FUNCTION_BLOCK FB_Visu
VAR
	// ============================== 轴 NCTOPLC 的输入结构体 =====================================
	
	// 这里没用AXIS_REF是因为轴变量不能多次绑定，而 NCTOPLC_AXIS_REF 的某些状态字是可以多次绑定的，在模拟程序中，只会用到一些状态字去检测轴的一些 NC 参数
	
	MainAxisState			AT %I*		: NCTOPLC_AXIS_REF;			// 运输皮带 	NCTOPLC 的输入结构体
	MetalAxisState			AT %I*		: NCTOPLC_AXIS_REF;			// 金属分拣皮带 NCTOPLC 的输入结构体
	PlasticAxisState		AT %I*		: NCTOPLC_AXIS_REF;			// 塑料分拣皮带 NCTOPLC 的输入结构体
	bresetAxis				AT %Q*      : BOOL;						// 如果主程序当中的轴出现 NC 报错，那需要在 HMI 当中做一个按钮去复位轴报错
	
	// =================================== 设备的一些状态 ===============================
	bComprAirEnabled		AT %I*		: BOOL;						// 如果为TRUE，则设备的气缸空气被压缩
	bPowerEnabled			AT %I*		: BOOL;						// 如果为TRUE，则设备已经使能
	bClampToWork			AT %I*		: BOOL;						// 如果为TRUE，则正位气缸存在输出
	bBarrierToWork			AT %I*		: BOOL;						// 如果为TRUE，则栏杆气缸存在输出
	bMetalToWork			AT %I*		: BOOL;						// 如果为TRUE，则金属分拣气缸存在输出
	bPlasticToWork			AT %I*		: BOOL;						// 如果为TRUE，则塑料分拣气缸存在输出
	
	// ====================================== 错误信息 ====================================
	bError					AT %I*		: BOOL;						// 如果为TRUE，则设备存在错误
	bClampError				AT %I*		: BOOL;						// 如果为TRUE，则正位气缸存在错误
	sClampErrMsg			AT %I*		: STRING;					// 正位气缸的错误信息
	bMetalCylError			AT %I*		: BOOL;						// 如果为TRUE，则金属分拣气缸存在错误
	sMetalErrMsg			AT %I*		: STRING;					// 金属分拣气缸的错误信息
	bPlasticCylError		AT %I*		: BOOL;						// 如果为TRUE，则塑料分拣气缸存在错误
	sPlasticErrMsg			AT %I*		: STRING;					// 塑料分拣气缸的错误信息
	sMessageMainAxis		AT %I*		: STRING;					// 运输皮带的错误信息
	sMessageMetalAxis		AT %I*		: STRING;					// 金属分拣出料皮带的错误信息
	sMessagePlasticAxis		AT %I*		: STRING;					// 塑料分拣出料皮带的错误信息

	
	// ============================ PackML状态机的状态标志位 ==============================
	bStarted				AT %I*		: BOOL;						// 如果为TRUE，则设备在运行状态
	bStopped				AT %I*		: BOOL;						// 如果为TRUE，则设备在停止状态
	bReset					AT %I*		: BOOL;						// 如果为TRUE，则设备在复位中状态
	bAborted				AT %I*		: BOOL;						// 如果为TRUE，则设备在中止状态
	bIdle					AT %I*		: BOOL;						// 如果为TRUE，则设备在空闲状态
	bAuto					AT %I*		: BOOL;						// 如果为TRUE，则设备在自动模式
	bSemi					AT %I*		: BOOL;						// 如果为TRUE，则设备在半自动模式
	bManual					AT %I*		: BOOL;						// 如果为TRUE，则设备在手动模式
	bMaintenance			AT %I*		: BOOL;						// 如果为TRUE，则设备在维护模式
	
	bStartButtonOff			AT %I*		: BOOL;						// 自复位启动按钮的中间变量

	// ============================ HMI 按钮输入的状态 ==================================
	
	// HMI按钮信号直接传递给bButtonXXXOut，绑定给主程序信号处理功能块的In，然后经过主程序信号处理功能块的Out绑定回来，用来做一些 HMI 按钮颜色，切换的逻辑
	
	bButtonPowerIn			AT %I*		: BOOL;						// 使能按钮的状态
	bButtonComprAirIn		AT %I*		: BOOL;						// 气缸压缩按钮的状态
	bButtonStartIn			AT %I*		: BOOL;						// 启动按钮的状态
	bButtonStopIn			AT %I*		: BOOL;						// 停止按钮的状态
	bButtonResetIn			AT %I*		: BOOL;						// 复位按钮的状态
	bButtonAbortIn			AT %I*		: BOOL;						// 中止按钮的状态
	
	bButtonAutoIn			AT %I*		: BOOL;						// 自动模式按钮的状态
	bButtonSemiIn			AT %I*		: BOOL;						// 半自动模式按钮的状态
	bButtonManuIn			AT %I*		: BOOL;						// 手动模式按钮的状态
	bButtonMaintenanceIn	AT %I*		: BOOL;						// 维护模式按钮的状态

	bButtonMainFwIn			AT %I*		: BOOL;						// 正向点动输送皮带按钮的状态
	bButtonMainBwIn			AT %I*		: BOOL;						// 反向点动输送皮带按钮的状态
	bButtonMetalFwIn		AT %I*		: BOOL;						// 正向点动金属分拣出料皮带按钮的状态
	bButtonMetalBwIn		AT %I*		: BOOL;						// 反向点动金属分拣出料皮带按钮的状态
	bButtonPlasticFwIn		AT %I*		: BOOL;						// 正向点动塑料分拣出料皮带按钮的状态
	bButtonPlasticBwIn		AT %I*		: BOOL;						// 反向点动塑料分拣出料皮带按钮的状态
	
	bButtonClampToWorkIn	AT %I*		: BOOL;						// 正位气缸输出按钮的状态
	bButtonBarrierToWorkIn	AT %I*		: BOOL;						// 栏杆气缸输出按钮的状态
	bButtonMetalToWorkIn	AT %I*		: BOOL;						// 金属分拣气缸输出按钮的状态
	bButtonPlasticToWorkIn	AT %I*		: BOOL;						// 塑料分拣气缸输出按钮的状态


	
	// ============================== HMI 按钮的输出信号 ===============================
	
	// 绑定给主程序信号处理功能块的In
	
	bButtonPowerOut			AT %Q*		: BOOL;						// 使能按钮的信号
	bButtonComprAirOut		AT %Q*		: BOOL;						// 气缸压缩按钮的信号
	bButtonStartOut			AT %Q*		: BOOL;						// 启动按钮的信号
	bButtonStopOut			AT %Q*		: BOOL;						// 停止按钮的信号
	bButtonResetOut			AT %Q*		: BOOL;						// 复位按钮的信号
	
	bButtonAutoOut			AT %Q*		: BOOL;						// 自动模式按钮的信号	
	bButtonSemiOut			AT %Q*		: BOOL;						// 半自动模式按钮的信号
	bButtonManuOut			AT %Q*		: BOOL;						// 手动模式按钮的信号
	bButtonMaintenanceOut	AT %Q*		: BOOL;						// 维护模式按钮的信号	
	
	bButtonMainFwOut		AT %Q*		: BOOL;						// 正向点动输送皮带按钮的信号
	bButtonMainBwOut		AT %Q*		: BOOL;						// 反向点动输送皮带按钮的信号
	bButtonMetalFwOut		AT %Q*		: BOOL;						// 正向点动金属分拣出料皮带按钮的信号
	bButtonMetalBwOut		AT %Q*		: BOOL;						// 反向点动金属分拣出料皮带按钮的信号
	bButtonPlasticFwOut		AT %Q*		: BOOL;						// 正向点动塑料分拣出料皮带按钮的信号
	bButtonPlasticBwOut		AT %Q*		: BOOL;						// 反向点动塑料分拣出料皮带按钮的信号
	
	bButtonClampToWorkOut	AT %Q*		: BOOL;						// 正位气缸输出按钮的信号
	bButtonBarrierToWorkOut	AT %Q*		: BOOL;						// 栏杆气缸输出按钮的信号
	bButtonMetalToWorkOut	AT %Q*		: BOOL;						// 金属分拣气缸输出按钮的信号
	bButtonPlasticToWorkOut	AT %Q*		: BOOL;						// 塑料分拣气缸输出按钮的信号

	
	// =========================== 模拟程序当中元素的坐标参数 ===========================
	fYClamp								: LREAL;					// 正位气缸的纵坐标
	fYBarrier							: LREAL;					// 栏杆气缸的纵坐标
	fYMetal								: LREAL;					// 金属分拣气缸的纵坐标
	fYPlastic							: LREAL;					// 塑料分拣气缸的纵坐标
	aBoxX								: ARRAY[1..4] OF LREAL;		// 物料的横坐标数组
	aBoxY								: ARRAY[1..4] OF LREAL;		// 物料的纵坐标数组

	// ============================= 物料移动参数 =========================================
	nLastBox						: INT;						// 在运输皮带当中物料的序号，			如：nLastBox := 1，则一号物料在运输当中
	aBoxMetalMove					: ARRAY[1..4] OF BOOL;		// 第几个物料在被金属分拣气缸分拣，		如：aBoxMetalMove[1] := TRUE，则一号物料在被金属分拣气缸分拣
	aBoxMetalFree					: ARRAY[1..4] OF BOOL;		// 第几个物料没在被金属分拣气缸分拣		如：aBoxMetalFree[1] := TRUE，则一号物料没有在被金属分拣气缸分拣
	aBoxPlasticMove					: ARRAY[1..4] OF BOOL;		// 第几个物料在被塑料分拣气缸分拣		如：aBoxPlasticMove[1] := TRUE，则一号物料在被金属分拣气缸分拣
	aBoxPlasticFree					: ARRAY[1..4] OF BOOL;		// 第几个物料没在被塑料分拣气缸分拣		如：aBoxPlasticFree[1] := TRUE，则一号物料没有在被塑料分拣气缸分拣
	aBoxMainBelt					: ARRAY[1..4] OF BOOL;		// 第几个物料在运输皮带当中运输			如：aBoxMainBelt[1] := TRUE，则一号物料在运输当中
	aBoxMetalBelt					: ARRAY[1..4] OF BOOL;		// 第几个物料在金属分拣皮带当中运出		如：aBoxMetalBelt[1] := TRUE，则一号物料在运输当中
	aBoxPlasticBelt					: ARRAY[1..4] OF BOOL;		// 第几个物料在塑料分拣皮带当中运出		如：aBoxPlasticBelt[1] := TRUE，则一号物料在运输当中
	
	fMainVelo						: LREAL;					// 运输皮带的转动速度
	fMetalVelo						: LREAL;					// 金属分拣皮带的转动速度
	fPlasticVelo					: LREAL;					// 塑料分拣皮带的转动速度
	
	bAccident						: BOOL;						// 如果为TRUE，则出现意外事故			如：撞机
	nState							: INT;						// 物料的索引							如：nState := 1，则当前是1号物料
	
	// ================================= 信息 ==========================================
	nMessages						: INT;						// 信息的个数
	sMessageClamp					: STRING;					// 正位气缸的信息
	sMessageMetalCyl				: STRING;					// 金属分拣气缸的信息
	sMessagePlasticCyl				: STRING;					// 塑料分拣气缸的信息

	
	// ============================= 轴运动的参数 =======================================
	nAngleMain						: INT;						// 输送皮带转动时旋转的角度（HMI）
	nAngleMetal						: INT;						// 金属分拣皮带转动时旋转的角度（HMI）
	nAnglePlastic					: INT;						// 塑料分拣皮带转动时旋转的角度（HMI）
	fbTimerMainAxis					: TON;						// 输送皮带转动时到 HMI 图标开始转动的计时器 TON 功能块 
	fbTimerMetalAxis				: TON;						// 金属分拣皮带转动时到 HMI 图标开始转动的计时器 TON 功能块 
	fbTimerPlasticAxis				: TON;						// 塑料分拣皮带转动时到 HMI 图标开始转动的计时器 TON 功能块 
	tMoveAxis						: TIME := T#0MS;			// 皮带转动时到 HMI 图标开始转动的延迟时间，这里随机设置一个40ms较短的时间

	// ========================= 按钮颜色的相关参数 ====================================
	nButtonColorStart				: DWORD;					// 启动按钮的颜色
	bButtonColorStart				: BOOL;						// 如果为TRUE，则切换启动按钮的颜色
	nButtonColorStop				: DWORD;					// 停止按钮的颜色
	bButtonColorStop				: BOOL;						// 如果为TRUE，则切换停止按钮的颜色
	nButtonColorReset				: DWORD;					// 复位按钮的颜色
	bButtonColorReset				: BOOL;						// 如果为TRUE，则切换停止按钮的颜色
	nButtonColorAuto				: DWORD;					// 自动模式按钮的颜色
	bButtonColorAuto				: BOOL;						// 如果为TRUE，则切换自动模式按钮的颜色
	nButtonColorSemi				: DWORD;					// 半自动模式按钮的颜色
	bButtonColorSemi				: BOOL;						// 如果为TRUE，则切换半自动模式按钮的颜色
	nButtonColorManu				: DWORD;					// 手动模式按钮的颜色
	bButtonColorManu				: BOOL;						// 如果为TRUE，则切换手动模式按钮的颜色
	nButtonColorMaint				: DWORD;					// 维护模式按钮的颜色
	bButtonColorMaint				: BOOL;						// 如果为TRUE，则切换维护模式按钮的颜色
	nButtonColorClamp				: DWORD;					// 手动控制正位气缸按钮的颜色
	bButtonColorClamp				: BOOL;						// 如果为TRUE，则切换手动控制正位气缸按钮的颜色
	nButtonColorBarrier				: DWORD;					// 手动控制栏杆气缸按钮的颜色
	bButtonColorBarrier				: BOOL;						// 如果为TRUE，则切换手动控制栏杆气缸按钮的颜色
	nButtonColorMetalCyl			: DWORD;					// 手动控制金属分拣气缸按钮的颜色
	bButtonColorMetalCyl			: BOOL;						// 如果为TRUE，则切换金属分拣气缸按钮的颜色
	nButtonColorPlasticCyl			: DWORD;					// 手动控制塑料分拣气缸按钮的颜色
	bButtonColorPlasticCyl			: BOOL;						// 如果为TRUE，则切换塑料分拣气缸按钮的颜色
	nButtonColorMainFw				: DWORD;					// 手动控制输送皮带正转按钮的颜色
	bButtonColorMainFw				: BOOL;						// 如果为TRUE，则切换手动控制输送皮带正转按钮的颜色
	nButtonColorMainBw				: DWORD;					// 手动控制输送皮带反转按钮的颜色
	bButtonColorMainBw				: BOOL;						// 如果为TRUE，则切换手动控制输送皮带反转按钮的颜色
	nButtonColorMetalFw				: DWORD;					// 手动控制金属分拣皮带正转按钮的颜色
	bButtonColorMetalFw				: BOOL;						// 如果为TRUE，则切换手动控制金属分拣皮带正转按钮的颜色
	nButtonColorMetalBw				: DWORD;					// 手动控制金属分拣皮带反转按钮的颜色
	bButtonColorMetalBw				: BOOL;						// 如果为TRUE，则切换手动控制金属分拣皮带反转按钮的颜色
	nButtonColorPlasticFw			: DWORD;					// 手动控制塑料分拣皮带正转按钮的颜色
	bButtonColorPlasticFw			: BOOL;						// 如果为TRUE，则切换 手动控制塑料分拣皮带正转按钮的颜色
	nButtonColorPlasticBw			: DWORD;					// 手动控制塑料分拣皮带反转按钮的颜色
	bButtonColorPlasticBw			: BOOL;						// 如果为TRUE，则切换手动控制塑料分拣皮带反转按钮的颜色
	nButtonColorComprAir			: DWORD;					// 压缩气缸空气按钮的颜色
	bButtonColorComprAir			: BOOL;						// 如果为TRUE，则切换压缩气缸空气按钮的颜色

	// ================================== 其他 =======================================
	RandomGenerator					: DRAND;					// 随机函数生成的功能块
	RandomNumber					: LREAL;					// 随机数（0-1）
	bRandomChangeColor				: BOOL;						// 如果为TRUE，则随机的切换物料颜色
	ArrChangeColor					: ARRAY[1..4] OF BOOL	:= [TRUE,FALSE,FALSE,TRUE];	// 物料的随机颜色：如：ArrChangeColor[1]:= true; 则1号物料是灰色
	
	bButtonColorAutoNew				: BOOL;						// 如果为TRUE，则当前控制模式为自动模式且无报错，用来启用 HMI 当中的自动按钮
	bButtonColorSemiNew				: BOOL;						// 如果为TRUE，则当前控制模式为半自动模式且无报错，用来启用 HMI 当中的半自动按钮
	bButtonColorManuNew				: BOOL;						// 如果为TRUE，则当前控制模式为手动模式且无报错，用来启用 HMI 当中的手动按钮
	bButtonColorMaintNew			: BOOL;						// 如果为TRUE，则当前控制模式为维护模式且无报错，用来启用 HMI 当中的维护按钮
END_VAR
VAR CONSTANT
	// ================================== 颜色 =======================================
	cYellow 									: DWORD	:= 16#00FFFF80;		// 黄色的ARGB对应的16进制值
	cGreen 										: DWORD	:= 16#0080FF00;		// 绿色的ARGB对应的16进制值
	cPink 										: DWORD	:= 16#00FF8080;		// 粉色的ARGB对应的16进制值
	
	// ============================ HMI图标移动参数 ===================================
	cVelocityDenominator						: LREAL := 250.0;			// 速度比例分母。HMI 图标旋转的速度是实际轴速度的一个比值。
	cAxisMovementSemiPlusAuto					: INT 	:= 2;				// 半自动和自动模式下，HMI 轴每个PLC周期的移动角度
	cAxisMovementManual							: INT 	:= 1;				// 手动模式下，HMI 轴每个PLC周期的移动角度
	cClampMovement								: LREAL := 0.1;				// 每个PLC周期正位气缸的移动量
	cBarrierMovement							: LREAL := 1.0;				// 每个PLC周期栏杆气缸的移动量
	cMetalPlasticCylMovement					: LREAL := 1.0;				// 每个PLC周期塑料/金属分拣气缸的移动量
	
	// ========================= HMI图标各个位置的标定参数 ============================
	cYClampCylStartPos							: LREAL := 0.0;				// 正位气缸的基始位置纵坐标
	cYClampCylEndPos							: LREAL := 3.0;				// 正位气缸的目标位置纵坐标
	cYBarrierCylStartPos						: LREAL := 0.0;				// 栏杆气缸的基始位置纵坐标
	cYBarrierCylEndPos							: LREAL := 63.0;			// 栏杆气缸的目标位置纵坐标
	cYMetalPlasticCylStartPos					: LREAL := 0.0;				// 金属/塑料分拣气缸的基始位置纵坐标
	cYMetalPlasticCylEndPos						: LREAL := -73.0;			// 金属/塑料分拣气缸的目标位置纵坐标
	
	// =========================== 物料宽度、距离参数 ==================================
	cBoxWidth									: LREAL := 60.0;			// HMI 当中物料的宽度
	cBarrierWidth								: LREAL := 30.0;			// HMI 当中栏杆气缸的宽度
	cDiffBarrierToStartOfMetalCyl				: LREAL := 191.0;			// HMI 当中从栏杆气缸到金属分拣气缸左侧位置的距离，单位为像素或实际测量单位
	cDiffBarrierToEndOfMetalCyl					: LREAL := 261.0;			// HMI 当中从栏杆气缸到金属分拣气缸右侧位置的距离，单位为像素或实际测量单位
	cDiffBarrierToStartOfPlasticCyl				: LREAL := 441.0;			// HMI 当中从栏杆气缸到塑料分拣气缸左侧位置的距离，单位为像素或实际测量单位
	cYMetalPlasticCylOnMainBelt					: LREAL := -9.0;			// HMI 当中金属和塑料分拣气缸到达主传送带时的位置纵坐标
	cYBoxesOnMetalPlasticBelt_min				: LREAL := -65.0;			// HMI 当中物料在金属或塑出料皮带上时的最小位置的纵坐标
	cYBoxesOnMetalPlasticBelt_max				: LREAL := -140.0;			// HMI 当中物料在金属或塑出料皮带上时的最大位置的纵坐标
	
	// ======================== 输送皮带当中物料的距离参数 ==============================
	cYforAllBoxesOnMainBelt						: LREAL := -5.0;			// HMI 当中物料在输送皮带上的纵坐标
	cYforAllBoxesNotOnMainBelt					: LREAL := -60.0;			// HMI 当中物料不在输送皮带上的纵坐标
	
	cYforAllBoxesStartPosMainBelt				: LREAL := 0.0;				// HMI 当中物料在输送皮带的第一个位置时的纵坐标
	cXforAllBoxesStartPosMainBelt				: LREAL := -240.0;			// HMI 当中物料在输送皮带的第一个位置时的横坐标
	cXforAllBoxesLastPossiblePosMainBelt		: LREAL := 461.0;			// HMI 当中物料在输送皮带上，可以移动到的最后位置横坐标
	
	cXforAllBoxesCorrectPushMetalCyl_min		: LREAL := 180;				// HMI 当中被金属分拣气缸推到金属出料皮带时，物料最小位置的横坐标
	cXforAllBoxesCorrectPushMetalCyl_max		: LREAL := 211;				// HMI 当中被金属分拣气缸推到金属出料皮带时，物料最大位置的横坐标
	cXforAllBoxesIncorrectPushMetalCyl_min		: LREAL := 131;				// HMI 当中被金属分拣气缸推出，但未推到金属出料皮带时，物料最小位置的横坐标
	cXforAllBoxesIncorrectPushMetalCyl_max		: LREAL := 261;				// HMI 当中被金属分拣气缸推出，但未推到金属出料皮带时，物料最大位置的横坐标
	
	cXforAllBoxesCorrectPushPlasticCyl_min		: LREAL := 430;				// MMI 当中被塑料分拣气缸推到塑料出料皮带时，物料最小位置的横坐标
	cXforAllBoxesCorrectPushPlasticCyl_max		: LREAL := 461;				// HMI 当中被塑料分拣气缸推到塑料出料皮带时，物料最大位置的横坐标
	cXforAllBoxesIncorrectPushPlasticCyl_min	: LREAL := 381;				// HMI 当中被塑料分拣气缸推出，但未推到塑料出料皮带时，物料最小位置的横坐标
	
	// Box 1
	cXforBox1_MainBelt_Diff2to1_min				: LREAL := 1;				// 物料 2 到物料 1 之间的最小距离，以便物料 1 能够在输送皮带上移动
	cXforBox1_MainBelt_Diff2to1_max				: LREAL := 121;				// 物料 2 到物料 1 之间的最大距离，以便物料 1 能够在输送皮带上移动 
	cXforBox1_MainBelt_Diff3to1_min				: LREAL := 61;				// 物料 3 到物料 1 之间的最小距离，以便物料 1 能够在输送皮带上移动（1+60）
	cXforBox1_MainBelt_Diff3to1_max				: LREAL := 181;				// 物料 3 到物料 1 之间的最大距离，以便物料 1 能够在输送皮带上移动
	cXforBox1_MainBelt_Diff4to1_min				: LREAL := 121;				// 物料 4 到物料 1 之间的最小距离，以便物料 1 能够在输送皮带上移动（1+120）
	cXforBox1_MainBelt_Diff4to1_max				: LREAL := 241;				// 物料 4 到物料 1 之间的最大距离，以便物料 1 能够在输送皮带上移动
	
	// Box 2
	cXforBox2_MainBelt_Diff1to2_min				: LREAL := -1;				// 物料 1 到物料 2 之间的最小距离，以便物料 2 能够在输送皮带上移动
	cXforBox2_MainBelt_Diff1to2_max				: LREAL := -121;			// 物料 1 到物料 2 之间的最大距离，以便物料 2 能够在输送皮带上移动
	cXforBox2_MainBelt_Diff3to2_min				: LREAL := 121;				// 物料 3 到物料 2 之间的最小距离，以便物料 2 能够在输送皮带上移动
	cXforBox2_MainBelt_Diff3to2_max				: LREAL := 1;				// 物料 3 到物料 2 之间的最小距离，以便物料 2 能够在输送皮带上移动
	cXforBox2_MainBelt_Diff4to2_min				: LREAL := 181;				// 物料 4 到物料 2 之间的最小距离，以便物料 2 能够在输送皮带上移动
	cXforBox2_MainBelt_Diff4to2_max				: LREAL := 61;				// 物料 4 到物料 2 之间的最小距离，以便物料 2 能够在输送皮带上移动

	// Box 3
	cXforBox3_MainBelt_Diff1to3_min				: LREAL := -61;				// 物料 1 到物料 3 之间的最小距离，以便物料 3 能够在输送皮带上移动
	cXforBox3_MainBelt_Diff1to3_max				: LREAL := -181;			// 物料 1 到物料 3 之间的最大距离，以便物料 3 能够在输送皮带上移动
	cXforBox3_MainBelt_Diff2to3_min				: LREAL := -1;				// 物料 2 到物料 3 之间的最小距离，以便物料 3 能够在输送皮带上移动
	cXforBox3_MainBelt_Diff2to3_max				: LREAL := -121;			// 物料 2 到物料 3 之间的最大距离，以便物料 3 能够在输送皮带上移动
	cXforBox3_MainBelt_Diff4to3_min				: LREAL := 121;				// 物料 4 到物料 3 之间的最小距离，以便物料 3 能够在输送皮带上移动
	cXforBox3_MainBelt_Diff4to3_max				: LREAL := 1;				// 物料 4 到物料 3 之间的最大距离，以便物料 3 能够在输送皮带上移动
	
	// Box 4
	cXforBox4_MainBelt_Diff1to4_min				: LREAL := -121;			// 物料 1 到物料 4 之间的最小距离，以便物料 4 能够在输送皮带上移动
	cXforBox4_MainBelt_Diff1to4_max				: LREAL := -241;			// 物料 1 到物料 4 之间的最大距离，以便物料 4 能够在输送皮带上移动
	cXforBox4_MainBelt_Diff2to4_min				: LREAL := -61;				// 物料 2 到物料 4 之间的最小距离，以便物料 4 能够在输送皮带上移动
	cXforBox4_MainBelt_Diff2to4_max				: LREAL := -181;			// 物料 2 到物料 4 之间的最大距离，以便物料 4 能够在输送皮带上移动
	cXforBox4_MainBelt_Diff3to4_min				: LREAL := -1;				// 物料 3 到物料 4 之间的最小距离，以便物料 4 能够在输送皮带上移动
	cXforBox4_MainBelt_Diff3to4_max				: LREAL := -121;			// 物料 4 到物料 4 之间的最大距离，以便物料 4 能够在输送皮带上移动
	
	// ========================= 金属分拣皮带当中物料的距离参数 ===========================
	// Box 1
	cXforBox1OnMetalBelt_min					: LREAL := 240;				// 物料 1 在金属分拣皮带上时位置的最小横坐标
	cXforBox1OnMetalBelt_max					: LREAL := 271;				// 物料 1 在金属分拣皮带上时位置的最大横坐标
	// Box 2
	cXforBox2OnMetalBelt_min					: LREAL := 300;				// 物料 2 在金属分拣皮带上时位置的最小横坐标
	cXforBox2OnMetalBelt_max					: LREAL := 331;				// 物料 2 在金属分拣皮带上时位置的最大横坐标
	// Box 3
	cXforBox3OnMetalBelt_min					: LREAL := 360;				// 物料 3 在金属分拣皮带上时位置的最小横坐标
	cXforBox3OnMetalBelt_max					: LREAL := 391;				// 物料 3 在金属分拣皮带上时位置的最大横坐标
	// Box 4
	cXforBox4OnMetalBelt_min					: LREAL := 420;				// 物料 4 在金属分拣皮带上时位置的最小横坐标
	cXforBox4OnMetalBelt_max					: LREAL := 451;				// 物料 4 在金属分拣皮带上时位置的最大横坐标
	
	// ========================= 塑料分拣皮带当中物料的距离参数 =========================
	// Box 1
	cXforBox1OnPlasticBelt_min					: LREAL := 470;				// 物料 1 在塑料分拣皮带上时位置的最小横坐标
	cXforBox1OnPlasticBelt_max					: LREAL := 521;				// 物料 1 在塑料分拣皮带上时位置的最大横坐标
	// Box 2
	cXforBox2OnPlasticBelt_min					: LREAL := 530;				// 物料 2 在塑料分拣皮带上时位置的最小横坐标
	cXforBox2OnPlasticBelt_max					: LREAL := 581;				// 物料 2 在塑料分拣皮带上时位置的最大横坐标
	// Box 3
	cXforBox3OnPlasticBelt_min					: LREAL := 590;				// 物料 3 在塑料分拣皮带上时位置的最小横坐标
	cXforBox3OnPlasticBelt_max					: LREAL := 641;				// 物料 3 在塑料分拣皮带上时位置的最大横坐标
	// Box 4
	cXforBox4OnPlasticBelt_min					: LREAL := 650;				// 物料 4 在塑料分拣皮带上时位置的最小横坐标
	cXforBox4OnPlasticBelt_max					: LREAL := 701;				// 物料 4 在塑料分拣皮带上时位置的最大横坐标
END_VAR

// =========================================================
// 复位
	
	IF bReset THEN
		Reset();
	END_IF
	
// =========================================================
// 出现事故立即切断使能
	
	IF bAccident THEN
		IF bButtonPowerOut THEN
			bButtonPowerOut := FALSE;
		END_IF
		
		IF bStopped THEN
			bAccident := FALSE;
		END_IF
	END_IF

// =========================================================
// 方法调用

	// 轴图标旋转
	AxisRotation();
	
	// 按钮信号、颜色、物料状态
	ButtonSignals();
	ButtonColors();
	LastBox();
	ErrorMessages();
	
	// 气缸移动
	Barrier_Clamp_Cyl();
	Metal_Plastic_Cyl();
	
	// 物料移动
	AxisMoveBoxes();
	CylinderMoveBoxes();
	
	// 随机刷新物料的颜色
	RandomColor();

// =========================================================
// 启用禁用模式按钮
    bButtonColorAutoNew                 := bButtonColorAuto  AND NOT bError;
	bButtonColorSemiNew                 := bButtonColorSemi  AND NOT bError;
	bButtonColorManuNew                 := bButtonColorManu  AND NOT bError; 
	bButtonColorMaintNew                := bButtonColorMaint AND NOT bError;

METHOD PRIVATE AxisMoveBoxes
VAR_INPUT
END_VAR
// ======================== 检测各个物料是否在输送皮带上的位置 =================================
		
	aBoxMainBelt[1] := 	// 物料 1 在输送皮带上
						aBoxY[1] >= cYforAllBoxesOnMainBelt											
						AND (	(aBoxX[2] - aBoxX[1] - fMainVelo) >= cXforBox1_MainBelt_Diff2to1_max
							OR 	(aBoxX[2] - aBoxX[1] - fMainVelo) <= cXforBox1_MainBelt_Diff2to1_min
							OR 	aBoxY[2] < cYforAllBoxesNotOnMainBelt)	
						AND (	(aBoxX[3] - aBoxX[1] - fMainVelo) >= cXforBox1_MainBelt_Diff3to1_max
							OR 	(aBoxX[3] - aBoxX[1]- fMainVelo) <= cXforBox1_MainBelt_Diff3to1_min
							OR 	aBoxY[3] < cYforAllBoxesNotOnMainBelt)
						AND (	(aBoxX[4] - aBoxX[1] - fMainVelo) >= cXforBox1_MainBelt_Diff4to1_max
							OR 	(aBoxX[4] - aBoxX[1]- fMainVelo) <= cXforBox1_MainBelt_Diff4to1_min
							OR	aBoxY[4] < cYforAllBoxesNotOnMainBelt);
						
	aBoxMainBelt[2] := 	// 物料 2 在输送皮带上
						aBoxY[2] >= cYforAllBoxesOnMainBelt										
						AND (	(aBoxX[1] - aBoxX[2] - fMainVelo) >= cXforBox2_MainBelt_Diff1to2_min 
							OR 	(aBoxX[1] - aBoxX[2] - fMainVelo) <= cXforBox2_MainBelt_Diff1to2_max 
							OR 	aBoxY[1] < cYforAllBoxesNotOnMainBelt)										
						AND (	(aBoxX[3] - aBoxX[2] - fMainVelo) >= cXforBox2_MainBelt_Diff3to2_min 
							OR 	(aBoxX[3] - aBoxX[2] - fMainVelo) <= cXforBox2_MainBelt_Diff3to2_max 
							OR 	aBoxY[3] < cYforAllBoxesNotOnMainBelt)									
						AND (	(aBoxX[4] - aBoxX[2] - fMainVelo) >= cXforBox2_MainBelt_Diff4to2_min 
							OR 	(aBoxX[4] - aBoxX[2] - fMainVelo) <= cXforBox2_MainBelt_Diff4to2_max 
							OR 	aBoxY[4] < cYforAllBoxesNotOnMainBelt);
	
	aBoxMainBelt[3] :=  // 物料 3 在输送皮带上
						aBoxY[3] >= cYforAllBoxesOnMainBelt											
						AND (	(aBoxX[1] - aBoxX[3] - fMainVelo) >= cXforBox3_MainBelt_Diff1to3_min
							OR 	(aBoxX[1] - aBoxX[3] - fMainVelo) <= cXforBox3_MainBelt_Diff1to3_max
							OR 	aBoxY[1] < cYforAllBoxesNotOnMainBelt)											
						AND (	(aBoxX[2] - aBoxX[3] - fMainVelo) >= cXforBox3_MainBelt_Diff2to3_min
							OR 	(aBoxX[2] - aBoxX[3] - fMainVelo) <= cXforBox3_MainBelt_Diff2to3_max 
							OR 	aBoxY[2] < cYforAllBoxesNotOnMainBelt)										
						AND (	(aBoxX[4] - aBoxX[3] - fMainVelo) >= cXforBox3_MainBelt_Diff4to3_min
							OR 	(aBoxX[4] - aBoxX[3] - fMainVelo) <= cXforBox3_MainBelt_Diff4to3_max
							OR 	aBoxY[4] < cYforAllBoxesNotOnMainBelt);
						
	aBoxMainBelt[4] := 	// 物料 4 在输送皮带上
						aBoxY[4] >= cYforAllBoxesOnMainBelt										
						AND (	(aBoxX[1] - aBoxX[4] - fMainVelo) >= cXforBox4_MainBelt_Diff1to4_min
							OR 	(aBoxX[1] - aBoxX[4] - fMainVelo) <= cXforBox4_MainBelt_Diff1to4_max
							OR 	aBoxY[1] < cYforAllBoxesNotOnMainBelt)										
						AND (	(aBoxX[2] - aBoxX[4] - fMainVelo) >= cXforBox4_MainBelt_Diff2to4_min
							OR 	(aBoxX[2] - aBoxX[4] - fMainVelo) <= cXforBox4_MainBelt_Diff2to4_max
							OR 	aBoxY[2] < cYforAllBoxesNotOnMainBelt)										
						AND (	(aBoxX[3] - aBoxX[4] - fMainVelo) >= cXforBox4_MainBelt_Diff3to4_min
							OR 	(aBoxX[3] - aBoxX[4] - fMainVelo) <= cXforBox4_MainBelt_Diff3to4_max
							OR 	aBoxY[3] < cYforAllBoxesNotOnMainBelt);
					
// ========================= 物料在皮带上的正向运动过程 ================================
		
	IF (NOT (BIT_TO_BOOL(MainAxisState.StateDWord.2))) AND (bAuto OR bSemi OR bButtonMainFwIn) THEN
		FOR nState := 1 TO 4 BY 1 DO
			
			IF aBoxMainBelt[nState] THEN	
				IF aBoxX[nState] >= (cBoxWidth*nState + cBarrierWidth) AND aBoxX[nState] < (cBoxWidth*nState + cDiffBarrierToEndOfMetalCyl - 1) THEN
					IF fYMetal <= cYMetalPlasticCylOnMainBelt THEN
						IF aBoxX[nState] < (cBoxWidth*nState + cDiffBarrierToStartOfMetalCyl - cBoxWidth + 0.25)
						AND aBoxX[nState] > (cBoxWidth*nState + cDiffBarrierToStartOfMetalCyl - cBoxWidth - 0.15) THEN
							aBoxX[nState] := cBoxWidth*nState + cDiffBarrierToStartOfMetalCyl - cBoxWidth;
						ELSIF aBoxX[nState] <= (cBoxWidth*nState + cDiffBarrierToStartOfMetalCyl - cBoxWidth - 0.15) THEN
							aBoxX[nState] := aBoxX[nState] + fMainVelo;
						END_IF
					ELSE
						aBoxX[nState] := aBoxX[nState] + fMainVelo;
					END_IF
				END_IF

				IF aBoxX[nState] >= (cBoxWidth*nState + cDiffBarrierToEndOfMetalCyl - 1) THEN
					IF fYPlastic <= cYMetalPlasticCylOnMainBelt THEN
						IF aBoxX[nState] < (cBoxWidth*nState + cDiffBarrierToStartOfPlasticCyl - cBoxWidth + 0.25)
						AND aBoxX[nState] > (cBoxWidth*nState + cDiffBarrierToStartOfPlasticCyl - cBoxWidth - 0.15) THEN
							aBoxX[nState] := cBoxWidth*nState + cDiffBarrierToStartOfPlasticCyl - cBoxWidth;
						ELSIF aBoxX[nState] <= (cBoxWidth*nState + cDiffBarrierToStartOfPlasticCyl - cBoxWidth - 0.15) THEN
							aBoxX[nState] := aBoxX[nState] + fMainVelo;
						END_IF
					ELSE
						aBoxX[nState] := aBoxX[nState] + fMainVelo;
					END_IF
				END_IF
				
				IF fYBarrier >= (cBoxWidth + 1) AND aBoxX[nState] >= cBoxWidth*(nState - 1) AND aBoxX[nState] <  (cBoxWidth*nState + cBarrierWidth) THEN
					IF aBoxX[nState] + fMainVelo < (cBoxWidth*nState + cBarrierWidth) THEN
						 aBoxX[nState] := aBoxX[nState] + fMainVelo;
					ELSIF aBoxX[nState] < (cBoxWidth*nState + cBarrierWidth) THEN
						aBoxX[nState] := (cBoxWidth*nState + cBarrierWidth);
					END_IF
				END_IF
				
				IF aBoxX[nState] + fMainVelo < -cBoxWidth*(3 - nState) THEN
					aBoxX[nState] := aBoxX[nState] + fMainVelo;
				ELSIF aBoxX[nState] < -cBoxWidth*(nState + 1) THEN
					aBoxX[nState] := -cBoxWidth*(nState + 1);
				END_IF
													
				IF fYClamp >= 1 AND aBoxX[nState] >= -cBoxWidth*(nState + 1) THEN
					IF aBoxX[nState] + fMainVelo < cBoxWidth*(nState - 1) THEN
						aBoxX[nState] := aBoxX[nState] + fMainVelo;
					ELSIF aBoxX[nState] < cBoxWidth*(nState - 1) THEN
						aBoxX[nState] := cBoxWidth*(nState - 1);
					END_IF
				END_IF
			END_IF
		END_FOR
	END_IF

// ========================= 物料在皮带上的反向运动过程 ================================
	
	IF (NOT (BIT_TO_BOOL(MainAxisState.StateDWord.2)))  AND bButtonMainBwIn THEN 
		FOR nState := 1 TO 4 BY 1 DO
			IF aBoxMainBelt[nState] THEN
				IF aBoxX[nState] >= (cBoxWidth*nState + cBoxWidth + cBarrierWidth) AND aBoxX[nState] < (cBoxWidth*nState + cDiffBarrierToEndOfMetalCyl + 1) THEN
					IF NOT (aBoxX[nState] < (cBoxWidth*nState + cDiffBarrierToEndOfMetalCyl + 0.25)
					AND aBoxX[nState] > (cBoxWidth*nState + cDiffBarrierToEndOfMetalCyl - 0.15)
					AND P_fYMetal <= cYMetalPlasticCylOnMainBelt) THEN
						aBoxX[nState] := aBoxX[nState] + fMainVelo;
					ELSE
						aBoxX[nState] := cBoxWidth*nState + cDiffBarrierToEndOfMetalCyl;
					END_IF
				END_IF

				IF aBoxX[nState] >= (cBoxWidth*nState + cDiffBarrierToEndOfMetalCyl + 1) THEN
					aBoxX[nState] := aBoxX[nState] + fMainVelo;
				END_IF

				IF aBoxX[nState] > cBoxWidth*(nState - 1) AND aBoxX[nState] < (cBoxWidth*nState + cBoxWidth + cBarrierWidth) THEN
					IF NOT (aBoxX[nState] < (cBoxWidth*nState + cBarrierWidth + 0.25)
					AND aBoxX[nState] > (cBoxWidth*nState + cBarrierWidth - 0.15)
					AND fYBarrier < (cBoxWidth + 1)) THEN
						aBoxX[nState] := aBoxX[nState] + fMainVelo;
					ELSE
						aBoxX[nState] := cBoxWidth*nState + cBarrierWidth;
					END_IF
				END_IF

				IF fYBarrier >= (cBoxWidth + 1) AND aBoxX[nState] < cBoxWidth*(nState + 1) AND aBoxX[nState] > cBoxWidth*(nState - 1) THEN
					aBoxX[nState] := aBoxX[nState] + fMainVelo;
				END_IF	
										
				IF fYClamp >= 1 AND aBoxX[nState] <= cBoxWidth*(nState-1) AND aBoxX[nState] > -cBoxWidth*(3-nState) THEN
					aBoxX[nState] := aBoxX[nState] + fMainVelo;
				END_IF
				
				IF aBoxX[nState] > -cBoxWidth*(4-nState) AND aBoxX[nState] <= -cBoxWidth*(3-nState) THEN
					aBoxX[nState] := aBoxX[nState] + fMainVelo;
				END_IF
			END_IF
		END_FOR	
	END_IF

// ===========================检测各个物料在金属出料皮带当中是否正在被运输==============================

	aBoxMetalBelt[1] := 
						aBoxX[1] > cXforBox1OnMetalBelt_min AND aBoxX[1] <= cXforBox1OnMetalBelt_max											
						AND ((aBoxY[2] - aBoxY[1] - fMetalVelo) >= cBoxWidth OR (aBoxY[2] - aBoxY[1] - fMetalVelo) <= -cBoxWidth
							OR NOT (aBoxX[2] > cXforBox2OnMetalBelt_min AND aBoxX[2] <= cXforBox2OnMetalBelt_max))
						AND ((aBoxY[3] - aBoxY[1]- fMetalVelo) >= cBoxWidth OR (aBoxY[3] - aBoxY[1]- fMetalVelo) <= -cBoxWidth
							OR NOT (aBoxX[3] > cXforBox3OnMetalBelt_min AND aBoxX[3] <= cXforBox3OnMetalBelt_max))
						AND ((aBoxY[4] - aBoxY[1]- fMetalVelo) >= cBoxWidth OR (aBoxY[4] - aBoxY[1]- fMetalVelo) <= -cBoxWidth
							OR NOT (aBoxX[4] > cXforBox4OnMetalBelt_min AND aBoxX[4] <= cXforBox4OnMetalBelt_max));	
						
	aBoxMetalBelt[2] := aBoxX[2] > cXforBox2OnMetalBelt_min AND aBoxX[2] <= cXforBox2OnMetalBelt_max										
						AND ((aBoxY[1] - aBoxY[2] - fMetalVelo) >= cBoxWidth OR (aBoxY[1] - aBoxY[2] - fMetalVelo) <= -cBoxWidth
							OR NOT (aBoxX[1] > cXforBox1OnMetalBelt_min AND aBoxX[1] <= cXforBox1OnMetalBelt_max))
						AND ((aBoxY[3] - aBoxY[2]- fMetalVelo) >= cBoxWidth OR (aBoxY[3] - aBoxY[2]- fMetalVelo) <= -cBoxWidth
							OR NOT (aBoxX[3] > cXforBox3OnMetalBelt_min AND aBoxX[3] <= cXforBox3OnMetalBelt_max))
						AND ((aBoxY[4] - aBoxY[2]- fMetalVelo) >= cBoxWidth OR (aBoxY[4] - aBoxY[2]- fMetalVelo) <= -cBoxWidth
							OR NOT (aBoxX[4] > cXforBox4OnMetalBelt_min AND aBoxX[4] <= cXforBox4OnMetalBelt_max));	
						
	aBoxMetalBelt[3] := aBoxX[3] > cXforBox3OnMetalBelt_min AND aBoxX[3] <= cXforBox3OnMetalBelt_max										
						AND ((aBoxY[1] - aBoxY[3] - fMetalVelo) >= cBoxWidth OR (aBoxY[1] - aBoxY[3] - fMetalVelo) <= -cBoxWidth
							OR NOT (aBoxX[1] > cXforBox1OnMetalBelt_min AND aBoxX[1] <= cXforBox1OnMetalBelt_max))
						AND ((aBoxY[2] - aBoxY[3]- fMetalVelo) >= cBoxWidth OR (aBoxY[2] - aBoxY[3]- fMetalVelo) <= -cBoxWidth
							OR NOT (aBoxX[2] > cXforBox2OnMetalBelt_min AND aBoxX[2] <= cXforBox2OnMetalBelt_max))
						AND ((aBoxY[4] - aBoxY[3]- fMetalVelo) >= cBoxWidth OR (aBoxY[4] - aBoxY[3]- fMetalVelo) <= -cBoxWidth
							OR NOT (aBoxX[4] > cXforBox4OnMetalBelt_min AND aBoxX[4] <= cXforBox4OnMetalBelt_max));	
						
	aBoxMetalBelt[4] := aBoxX[4] > cXforBox4OnMetalBelt_min AND aBoxX[4] <= cXforBox4OnMetalBelt_max										
						AND ((aBoxY[1] - aBoxY[4] - fMetalVelo) >= cBoxWidth OR (aBoxY[1] - aBoxY[4] - fMetalVelo) <= -cBoxWidth
							OR NOT (aBoxX[1] > cXforBox1OnMetalBelt_min AND aBoxX[1] <= cXforBox1OnMetalBelt_max))
						AND ((aBoxY[2] - aBoxY[4] - fMetalVelo) >= cBoxWidth OR (aBoxY[2] - aBoxY[4] - fMetalVelo) <= -cBoxWidth
							OR NOT (aBoxX[2] > cXforBox2OnMetalBelt_min AND aBoxX[2] <= cXforBox2OnMetalBelt_max))
						AND ((aBoxY[3] - aBoxY[4]- fMetalVelo) >= cBoxWidth OR (aBoxY[3] - aBoxY[4]- fMetalVelo) <= -cBoxWidth
							OR NOT (aBoxX[3] > cXforBox3OnMetalBelt_min AND aBoxX[3] <= cXforBox3OnMetalBelt_max));
// =========================================================
// 被分拣出料完成之后，回到初始位置、刷新随机颜色

		FOR nState := 1 TO 4 BY 1 DO	
		IF(NOT (BIT_TO_BOOL(MetalAxisState.StateDWord.2)))  THEN
			IF 	aBoxMetalBelt[nState] THEN
					IF bAuto OR bSemi OR (NOT bAuto AND bButtonMetalFwIn) THEN	
						IF aBoxY[nState] <= (cYBoxesOnMetalPlasticBelt_min + 0.1) AND aBoxY[nState] > cYBoxesOnMetalPlasticBelt_max THEN
							aBoxY[nState] := aBoxY[nState] + fMetalVelo;
						END_IF
						
					ELSIF NOT bAuto AND bButtonMetalBwIn THEN
						IF aBoxY[nState] + fMetalVelo <= (cYBoxesOnMetalPlasticBelt_min - 0.1) THEN
							aBoxY[nState] := aBoxY[nState] + fMetalVelo;
						END_IF
					END_IF
			END_IF
		END_IF	
		
		IF aBoxY[nState] <= (cYBoxesOnMetalPlasticBelt_max  )AND nLastBox = 0 THEN
			aBoxY[nState] := cYforAllBoxesStartPosMainBelt;
			aBoxX[nState] := cXforAllBoxesStartPosMainBelt + nState*cBoxWidth;
			IF bRandomChangeColor THEN
				ArrChangeColor[nState]	:= TRUE;
			ELSE
				ArrChangeColor[nState]	:= FALSE;
			END_IF
		END_IF

	END_FOR


// ===========================检测各个物料在塑料出料皮带当中是否正在被运输==============================
	
	aBoxPlasticBelt[1] := aBoxX[1] > cXforBox1OnPlasticBelt_min AND aBoxX[1] <= cXforBox1OnPlasticBelt_max											
						AND ((aBoxY[2] - aBoxY[1] - fPlasticVelo) >= cBoxWidth OR (aBoxY[2] - aBoxY[1] - fPlasticVelo) <= -cBoxWidth
								OR NOT (aBoxX[2] > cXforBox2OnPlasticBelt_min AND aBoxX[2] <= cXforBox2OnPlasticBelt_max))
						AND ((aBoxY[3] - aBoxY[1]- fPlasticVelo) >= cBoxWidth OR (aBoxY[3] - aBoxY[1]- fPlasticVelo) <= -cBoxWidth
								OR NOT (aBoxX[3] > cXforBox3OnPlasticBelt_min AND aBoxX[3] <= cXforBox3OnPlasticBelt_max))
						AND ((aBoxY[4] - aBoxY[1]- fPlasticVelo) >= cBoxWidth OR (aBoxY[4] - aBoxY[1]- fPlasticVelo) <= -cBoxWidth
								OR NOT (aBoxX[4] > cXforBox4OnPlasticBelt_min AND aBoxX[4] <= cXforBox4OnPlasticBelt_max));	
						
	aBoxPlasticBelt[2] := aBoxX[2] > cXforBox2OnPlasticBelt_min AND aBoxX[2] <= cXforBox2OnPlasticBelt_max									
						AND ((aBoxY[1] - aBoxY[2] - fPlasticVelo) >= cBoxWidth OR (aBoxY[1] - aBoxY[2] - fPlasticVelo) <= -cBoxWidth
								OR NOT (aBoxX[1] > cXforBox1OnPlasticBelt_min AND aBoxX[1] <= cXforBox1OnPlasticBelt_max))
						AND ((aBoxY[3] - aBoxY[2]- fPlasticVelo) >= cBoxWidth OR (aBoxY[3] - aBoxY[2]- fPlasticVelo) <= -cBoxWidth
								OR NOT (aBoxX[3] > cXforBox3OnPlasticBelt_min AND aBoxX[3] <= cXforBox3OnPlasticBelt_max))
						AND ((aBoxY[4] - aBoxY[2]- fPlasticVelo) >= cBoxWidth OR (aBoxY[4] - aBoxY[2]- fPlasticVelo) <= -cBoxWidth
								OR NOT (aBoxX[4] > cXforBox4OnPlasticBelt_min AND aBoxX[4] <= cXforBox4OnPlasticBelt_max));	
						
	aBoxPlasticBelt[3] := aBoxX[3] > cXforBox3OnPlasticBelt_min AND aBoxX[3] <= cXforBox3OnPlasticBelt_max										
						AND ((aBoxY[1] - aBoxY[3] - fPlasticVelo) >= cBoxWidth OR (aBoxY[1] - aBoxY[3] - fPlasticVelo) <= -cBoxWidth
								OR NOT (aBoxX[1] > cXforBox1OnPlasticBelt_min AND aBoxX[1] <= cXforBox1OnPlasticBelt_max))
						AND ((aBoxY[2] - aBoxY[3]- fPlasticVelo) >= cBoxWidth OR (aBoxY[2] - aBoxY[3]- fPlasticVelo) <= -cBoxWidth
								OR NOT (aBoxX[2] > cXforBox2OnPlasticBelt_min AND aBoxX[2] <= cXforBox2OnPlasticBelt_max))
						AND ((aBoxY[4] - aBoxY[3]- fPlasticVelo) >= cBoxWidth OR (aBoxY[4] - aBoxY[3]- fPlasticVelo) <= -cBoxWidth
								OR NOT (aBoxX[4] > cXforBox4OnPlasticBelt_min AND aBoxX[4] <= cXforBox4OnPlasticBelt_max));	
						
	aBoxPlasticBelt[4] := aBoxX[4] > cXforBox4OnPlasticBelt_min AND aBoxX[4] <= cXforBox4OnPlasticBelt_max										
						AND ((aBoxY[1] - aBoxY[4] - fPlasticVelo) >= cBoxWidth OR (aBoxY[1] - aBoxY[4] - fPlasticVelo) <= -cBoxWidth
								OR NOT (aBoxX[1] > cXforBox1OnPlasticBelt_min AND aBoxX[1] <= cXforBox1OnPlasticBelt_max))
						AND ((aBoxY[2] - aBoxY[4] - fPlasticVelo) >= cBoxWidth OR (aBoxY[2] - aBoxY[4] - fPlasticVelo) <= -cBoxWidth
								OR NOT (aBoxX[2] > cXforBox2OnPlasticBelt_min AND aBoxX[2] <= cXforBox2OnPlasticBelt_max))
						AND ((aBoxY[3] - aBoxY[4]- fPlasticVelo) >= cBoxWidth OR (aBoxY[3] - aBoxY[4]- fPlasticVelo) <= -cBoxWidth
								OR NOT (aBoxX[3] > cXforBox3OnPlasticBelt_min AND aBoxX[3] <= cXforBox3OnPlasticBelt_max));

// =========================================================
// 被分拣出料完成之后，回到初始位置、刷新随机颜色

	FOR nState := 1 TO 4 BY 1 DO	
		IF (NOT (BIT_TO_BOOL(PlasticAxisState.StateDWord.2)))  THEN
				IF 	aBoxPlasticBelt[nState] THEN	
					IF bAuto OR bSemi OR (NOT bAuto AND bButtonPlasticFwIn) THEN
						IF aBoxY[nState] <= (cYBoxesOnMetalPlasticBelt_min + 0.1) AND aBoxY[nState] > cYBoxesOnMetalPlasticBelt_max THEN
							aBoxY[nState] := aBoxY[nState] + fPlasticVelo;
						END_IF
						
					ELSIF NOT bAuto AND bButtonPlasticBwIn THEN
						IF aBoxY[nState] + fPlasticVelo <= (cYBoxesOnMetalPlasticBelt_min - 0.1) THEN
							aBoxY[nState] := aBoxY[nState] + fPlasticVelo;
						END_IF
					END_IF
				END_IF
		END_IF
		
		IF aBoxY[nState] <= cYBoxesOnMetalPlasticBelt_max AND nLastBox = 0 THEN
			aBoxY[nState] := cYforAllBoxesStartPosMainBelt;
			aBoxX[nState] := cXforAllBoxesStartPosMainBelt + nState*cBoxWidth;
			IF bRandomChangeColor THEN
				ArrChangeColor[nState]	:= TRUE;
			ELSE
				ArrChangeColor[nState]	:= FALSE;
			END_IF
						 
		END_IF
	END_FOR

// =========================================================
END_METHOD

METHOD PRIVATE AxisRotation
VAR_INPUT
END_VAR
// =========================================================
// 换算轴图标的旋转速度：实际速度/固定常数
	
	IF bAuto OR bSemi OR bButtonMainFwIn THEN
		fMainVelo := ( MainAxisState.ActVelo / cVelocityDenominator);
	ELSIF bButtonMainBwIn THEN
		fMainVelo := -( MainAxisState.ActVelo / cVelocityDenominator);
	END_IF
	
	IF bAuto OR bSemi OR bButtonMetalFwIn THEN
		fMetalVelo := -( MainAxisState.ActVelo / cVelocityDenominator);
	ELSIF bButtonMetalBwIn THEN
		fMetalVelo := ( MainAxisState.ActVelo / cVelocityDenominator);
	END_IF
	
	IF bAuto OR bSemi OR bButtonPlasticFwIn THEN
		fPlasticVelo := -( MainAxisState.ActVelo / cVelocityDenominator);
	ELSIF bButtonPlasticBwIn THEN
		fPlasticVelo := ( MainAxisState.ActVelo / cVelocityDenominator);
	END_IF

// =========================================================
// 输送皮带上轴 HMI 图标的运动
		
		IF (bAuto OR bSemi) AND (NOT (((BIT_TO_BOOL(MainAxisState.StateDWord.2)= TRUE))))THEN
			nAngleMain := nAngleMain + cAxisMovementSemiPlusAuto;
			
		ELSIF bButtonMainFwIn THEN
			nAngleMain := nAngleMain + cAxisMovementManual;
			
		ELSIF bButtonMainBwIn THEN
			nAngleMain := nAngleMain - cAxisMovementManual;
			
		ELSIF ((BIT_TO_BOOL(MainAxisState.StateDWord.2)= TRUE)) THEN
			nAngleMain := nAngleMain ;
		END_IF

// =========================================================
// 金属分拣皮带上轴 HMI 图标的运动
		
		IF (bAuto OR bSemi) AND (NOT (((BIT_TO_BOOL(MetalAxisState.StateDWord.2)= TRUE)))) THEN
			nAngleMetal := nAngleMetal + cAxisMovementSemiPlusAuto;
			
		ELSIF bButtonMetalFwIn THEN
			nAngleMetal := nAngleMetal + cAxisMovementManual;
			
		ELSIF bButtonMetalBwIn THEN
			nAngleMetal := nAngleMetal - cAxisMovementManual;
			
		ELSIF ((BIT_TO_BOOL(MetalAxisState.StateDWord.2)= TRUE)) THEN
			nAngleMetal := nAngleMetal ;
		END_IF

// =========================================================
// 塑料分拣皮带上轴 HMI 图标的运动
		
		IF (bAuto OR bSemi) AND (NOT (((BIT_TO_BOOL(PlasticAxisState.StateDWord.2)= TRUE)))) THEN
			nAnglePlastic := nAnglePlastic + cAxisMovementSemiPlusAuto;
			
		ELSIF bButtonPlasticFwIn THEN
			nAnglePlastic := nAnglePlastic + cAxisMovementManual;
			
		ELSIF bButtonPlasticBwIn THEN
			nAnglePlastic := nAnglePlastic - cAxisMovementManual;
			
		ELSIF ((BIT_TO_BOOL(PlasticAxisState.StateDWord.2)= TRUE)) THEN
			nAnglePlastic := nAnglePlastic ;
		END_IF

// =========================================================
END_METHOD

METHOD PRIVATE Barrier_Clamp_Cyl
VAR_INPUT
END_VAR
// =========================================================
// 移动正位气缸
	
	IF bClampToWork THEN
		IF (fYClamp + cClampMovement) < cYClampCylEndPos THEN
			fYClamp := fYClamp + cClampMovement;
		ELSE
			fYClamp := cYClampCylEndPos;
		END_IF
		
	ELSE
		IF (fYClamp - cClampMovement) > cYClampCylStartPos THEN
			fYClamp := fYClamp - cClampMovement;
		ELSE
			fYClamp := cYClampCylStartPos;
		END_IF
	END_IF

// =========================================================
// =========================================================
// 移动栏杆气缸
	
	IF bBarrierToWork THEN
		IF (fYBarrier + cBarrierMovement) < cYBarrierCylEndPos THEN
			fYBarrier := fYBarrier + cBarrierMovement;
		ELSE
			fYBarrier := cYBarrierCylEndPos;
		END_IF
		
	ELSE
		IF (fYBarrier - cBarrierMovement) > cYBarrierCylStartPos THEN
			fYBarrier := fYBarrier - cBarrierMovement;
		ELSE
			fYBarrier := cYBarrierCylStartPos;
		END_IF
	END_IF

// =========================================================
// 检测物料与气缸的位置是否重叠，检测事故发生
	
	IF fYBarrier <= cBoxWidth AND NOT bBarrierToWork THEN
		FOR nState := 1 TO 4 BY 1 DO
			IF aBoxX[nState] > (-cBoxWidth + 0.11 + cBoxWidth*nState) AND aBoxX[nState] < (cBoxWidth*nState + cBarrierWidth) AND aBoxY[nState] = 0
			AND NOT bStopped THEN
				bAccident := TRUE;
			END_IF
		END_FOR
	END_IF

// =========================================================
END_METHOD

METHOD PRIVATE ButtonColors
VAR_INPUT
END_VAR
// ========================== 启动按钮颜色 ===============================

// 选择模式之后		
	IF (bAccident OR (bPowerEnabled AND (NOT bStarted OR (bSemi AND bStarted))
		AND NOT bButtonStopIn AND NOT bButtonAbortIn AND NOT bButtonResetIn
		AND (bAuto OR bSemi OR bManual OR bMaintenance))) AND NOT (bError AND bIdle) THEN
		
			IF bButtonStartOut THEN
				nButtonColorStart := cGreen;			// 按下则按钮是绿色
			ELSE
				nButtonColorStart := cYellow;			// 未按下则按钮是黄色
			END_IF
			
			bButtonColorStart := TRUE;
	ELSE
		bButtonColorStart := FALSE;
	END_IF

// ========================== 停止按钮颜色 ===============================

// 选择模式之后		
	IF (bStarted OR bIdle) AND (bAuto OR bSemi OR bManual OR bMaintenance) THEN
		IF bButtonStopOut THEN
			nButtonColorStop := cGreen;					// 按下则按钮是绿色
		ELSE
			nButtonColorStop := cYellow;				// 未按下则按钮是黄色
		END_IF
		
		bButtonColorStop := TRUE;
	ELSE
		bButtonColorStop := FALSE;
	END_IF

// ========================== 复位按钮颜色 ===============================

// 出现停机或者重新上使能之后		
	IF bStopped AND bPowerEnabled THEN
		IF bButtonResetOut THEN
			nButtonColorReset := cGreen;				// 按下则按钮是绿色
		ELSE
			nButtonColorReset := cYellow;				// 未按下则按钮是黄色
		END_IF
		
		bButtonColorReset := TRUE;
	ELSE
		bButtonColorReset := FALSE;
	END_IF

// ========================== 模式按钮颜色 ===============================

// 使能之后，各个模式的按钮都变为黄色，按下对应的模式按钮之后，变成绿色	
	IF bPowerEnabled THEN
		IF NOT bAuto THEN
			IF bIdle THEN
				nButtonColorAuto 	:= cYellow;
				bButtonColorAuto 	:= TRUE;
			ELSE
				bButtonColorAuto 	:= FALSE;
			END_IF
		ELSE
			nButtonColorAuto 		:= cGreen;
			bButtonColorAuto 		:= TRUE;
		END_IF
		
		IF NOT bSemi THEN
			IF bIdle THEN
				nButtonColorSemi 	:= cYellow;
				bButtonColorSemi 	:= TRUE;
			ELSE
				bButtonColorSemi 	:= FALSE;
			END_IF
		ELSE
			nButtonColorSemi 		:= cGreen;
			bButtonColorSemi 		:= TRUE;
		END_IF
		
		IF NOT bManual THEN
			IF bIdle THEN
				nButtonColorManu 	:= cYellow;
				bButtonColorManu 	:= TRUE;
			ELSE
				bButtonColorManu 	:= FALSE;
			END_IF
		ELSE
			nButtonColorManu 		:= cGreen;
			bButtonColorManu 		:= TRUE;
		END_IF
		
		IF NOT bMaintenance THEN
			IF bIdle THEN
				nButtonColorMaint 	:= cYellow;
				bButtonColorMaint 	:= TRUE;
			ELSE
				bButtonColorMaint 	:= FALSE;
			END_IF
		ELSE
			nButtonColorMaint 		:= cGreen;
			bButtonColorMaint 		:= TRUE;
		END_IF
	END_IF

// ========================= 手动控制气缸和皮带的按钮 ================================

// 在手动或者维护模式下			
	IF (bManual OR bMaintenance) AND bStarted THEN
		
		// 气缸到目标位置，则按钮变为粉色。基始位置为黄色
		IF bButtonClampToWorkOut THEN
			nButtonColorClamp 	:= cPink;
		ELSE
			nButtonColorClamp 	:= cYellow;
		END_IF
		
		IF bButtonBarrierToWorkOut THEN
			nButtonColorBarrier := cPink;
		ELSE
			nButtonColorBarrier := cYellow;
		END_IF
		
		IF bButtonMetalToWorkOut THEN
			nButtonColorMetalCyl := cPink;
		ELSE
			nButtonColorMetalCyl := cYellow;
		END_IF
		
		IF bButtonPlasticToWorkOut THEN
			nButtonColorPlasticCyl := cPink;
		ELSE
			nButtonColorPlasticCyl := cYellow;
		END_IF
		
		bButtonColorClamp 		:= TRUE;
		bButtonColorBarrier 	:= TRUE;
		bButtonColorMetalCyl 	:= TRUE;
		bButtonColorPlasticCyl 	:= TRUE;
		
	// 轴正转，则正转按钮为粉色，否则为黄色。轴反转，则反转按钮为粉色，否则为黄色。
		IF bButtonMainBwOut THEN
			nButtonColorMainBw := cPink;
		ELSE
			nButtonColorMainBw := cYellow;
		END_IF
		
		IF bButtonMainFwOut THEN
			nButtonColorMainFw := cPink;
		ELSE
			nButtonColorMainFw := cYellow;
		END_IF
		
		IF bButtonMetalBwOut THEN
			nButtonColorMetalBw := cPink;
		ELSE
			nButtonColorMetalBw := cYellow;
		END_IF
		
		IF bButtonMetalFwOut THEN
			nButtonColorMetalFw := cPink;
		ELSE
			nButtonColorMetalFw := cYellow;
		END_IF
		
		IF bButtonPlasticBwOut THEN
			nButtonColorPlasticBw := cPink;
		ELSE
			nButtonColorPlasticBw := cYellow;
		END_IF
		
		IF bButtonPlasticFwOut THEN
			nButtonColorPlasticFw := cPink;
		ELSE
			nButtonColorPlasticFw := cYellow;
		END_IF
		
		bButtonColorMainBw 		:= NOT bButtonMainFwOut;
		bButtonColorMainFw 		:= NOT bButtonMainBwOut;
		bButtonColorMetalBw 	:= NOT bButtonMetalFwOut;
		bButtonColorMetalFw 	:= NOT bButtonMetalBwOut;
		bButtonColorPlasticBw 	:= NOT bButtonPlasticFwOut;
		bButtonColorPlasticFw 	:= NOT bButtonPlasticBwOut;
	ELSE
		bButtonColorClamp 		:= FALSE;
		bButtonColorBarrier 	:= FALSE;
		bButtonColorMetalCyl 	:= FALSE;
		bButtonColorPlasticCyl 	:= FALSE;
		bButtonColorMainBw 		:= FALSE;
		bButtonColorMainFw 		:= FALSE;
		bButtonColorMetalBw 	:= FALSE;
		bButtonColorMetalFw 	:= FALSE;
		bButtonColorPlasticBw 	:= FALSE;
		bButtonColorPlasticFw 	:= FALSE;
	END_IF
		
// =========================手动压缩气缸空气按钮================================

// 维护模式下			
	IF bMaintenance AND bStarted THEN
		IF bButtonComprAirIn THEN
			nButtonColorComprAir := cGreen;				// 按下则按钮是绿色
		ELSE
			nButtonColorComprAir := cYellow;			// 未按下则按钮是黄色
		END_IF
		
		bButtonColorComprAir := TRUE;
	ELSE
		bButtonColorComprAir := FALSE;
	END_IF

// =========================================================
END_METHOD

METHOD PRIVATE ButtonSignals
VAR_INPUT
END_VAR
// =========================================================
// 请求按钮根据实际状态自复位

	IF bStartButtonOff THEN
		bButtonStartOut := FALSE;
	END_IF
	
	IF bStopped THEN
		bButtonStopOut := FALSE;
	END_IF
	
	IF bReset THEN
		bButtonResetOut := FALSE;
	END_IF
	
	IF bManual THEN
		bButtonManuOut := FALSE;
	END_IF
	
	IF bAuto THEN
		bButtonAutoOut := FALSE;
	END_IF
	
	IF bSemi THEN
		bButtonSemiOut := FALSE;
	END_IF
	
	IF bMaintenance THEN
		bButtonMaintenanceOut := FALSE;
	END_IF

// =========================================================
END_METHOD

METHOD PRIVATE CylinderMoveBoxes
VAR_INPUT
END_VAR
// =========================================================
// 金属分拣气缸，检测物料在金属皮带上的位置
// 检测第几个物料没在被金属分拣气缸分拣		如：aBoxMetalFree[1] := TRUE，则一号物料没有在被金属分拣气缸分拣
	
	aBoxMetalFree[1] := 	NOT (aBoxX[2] > cXforBox2OnMetalBelt_min AND aBoxX[2] <= cXforBox2OnMetalBelt_max AND (aBoxY[1] - aBoxY[2]) <= (cBoxWidth + 1))
						AND NOT (aBoxX[3] > cXforBox3OnMetalBelt_min AND aBoxX[3] <= cXforBox3OnMetalBelt_max AND (aBoxY[1] - aBoxY[3]) <= (cBoxWidth + 1))
						AND NOT (aBoxX[4] > cXforBox4OnMetalBelt_min AND aBoxX[4] <= cXforBox4OnMetalBelt_max AND (aBoxY[1] - aBoxY[4]) <= (cBoxWidth + 1));
	
	aBoxMetalFree[2] := 	NOT (aBoxX[1] > cXforBox1OnMetalBelt_min AND aBoxX[1] <= cXforBox1OnMetalBelt_max AND (aBoxY[2] - aBoxY[1]) <= (cBoxWidth + 1))
						AND NOT (aBoxX[3] > cXforBox3OnMetalBelt_min AND aBoxX[3] <= cXforBox3OnMetalBelt_max AND (aBoxY[2] - aBoxY[3]) <= (cBoxWidth + 1))
						AND NOT (aBoxX[4] > cXforBox4OnMetalBelt_min AND aBoxX[4] <= cXforBox4OnMetalBelt_max AND (aBoxY[2] - aBoxY[4]) <= (cBoxWidth + 1));
						
	aBoxMetalFree[3] := 	NOT (aBoxX[1] > cXforBox1OnMetalBelt_min AND aBoxX[1] <= cXforBox1OnMetalBelt_max AND (aBoxY[3] - aBoxY[1]) <= (cBoxWidth + 1))
						AND NOT (aBoxX[2] > cXforBox2OnMetalBelt_min AND aBoxX[2] <= cXforBox2OnMetalBelt_max AND (aBoxY[3] - aBoxY[2]) <= (cBoxWidth + 1))
						AND NOT (aBoxX[4] > cXforBox4OnMetalBelt_min AND aBoxX[4] <= cXforBox4OnMetalBelt_max AND (aBoxY[3] - aBoxY[4]) <= (cBoxWidth + 1));
						
	aBoxMetalFree[4] := 	NOT (aBoxX[1] > cXforBox1OnMetalBelt_min AND aBoxX[1] <= cXforBox1OnMetalBelt_max AND (aBoxY[4] - aBoxY[1]) <= (cBoxWidth + 1))
						AND NOT (aBoxX[2] > cXforBox2OnMetalBelt_min AND aBoxX[2] <= cXforBox2OnMetalBelt_max AND (aBoxY[4] - aBoxY[2]) <= (cBoxWidth + 1))
						AND NOT (aBoxX[3] > cXforBox3OnMetalBelt_min AND aBoxX[3] <= cXforBox3OnMetalBelt_max AND (aBoxY[4] - aBoxY[3]) <= (cBoxWidth + 1));

// =========================================================
// 金属分拣气缸移动金属物料
	
	FOR nState := 1 TO 4 BY 1 DO
		IF bMetalToWork AND aBoxMetalMove[nState] AND aBoxMetalFree[nState] THEN
			IF (fYMetal - cMetalPlasticCylMovement) >= (cYMetalPlasticCylEndPos + cMetalPlasticCylMovement) THEN
				fYMetal := fYMetal - cMetalPlasticCylMovement;
				
				IF (fYMetal - aBoxY[nState]) <= cYMetalPlasticCylOnMainBelt THEN
					aBoxY[nState] := aBoxY[nState] - cMetalPlasticCylMovement;
				END_IF
				
			ELSIF fYMetal = (cYMetalPlasticCylEndPos + cMetalPlasticCylMovement) AND (fYMetal - aBoxY[nState]) <= cYMetalPlasticCylOnMainBelt THEN
				aBoxY[nState] := aBoxY[nState] - 2*cMetalPlasticCylMovement;
				
			ELSE
				aBoxMetalMove[nState] := FALSE;
			END_IF
		END_IF	
	END_FOR

// =========================================================
// 塑料分拣气缸，检测物料在塑料皮带上的位置
// 检测第几个物料没在被塑料分拣气缸分拣		如：aBoxPlasticFree[1] := TRUE，则一号物料没有在被塑料分拣气缸分拣

	aBoxPlasticFree[1] := 	NOT (aBoxX[2] > (cXforBox2OnPlasticBelt_min + 20) AND aBoxX[2] <= cXforBox2OnPlasticBelt_max AND (aBoxY[1] - aBoxY[2]) <= (cBoxWidth + 1))
						AND NOT (aBoxX[3] > (cXforBox3OnPlasticBelt_min + 20) AND aBoxX[3] <= cXforBox3OnPlasticBelt_max AND (aBoxY[1] - aBoxY[3]) <= (cBoxWidth + 1))
						AND NOT (aBoxX[4] > (cXforBox4OnPlasticBelt_min + 20) AND aBoxX[4] <= cXforBox4OnPlasticBelt_max AND (aBoxY[1] - aBoxY[4]) <= (cBoxWidth + 1));
	
	aBoxPlasticFree[2] := 	NOT (aBoxX[1] > (cXforBox1OnPlasticBelt_min + 20) AND aBoxX[1] <= cXforBox1OnPlasticBelt_max AND (aBoxY[2] - aBoxY[1]) <= (cBoxWidth + 1))
						AND NOT (aBoxX[3] > (cXforBox3OnPlasticBelt_min + 20) AND aBoxX[3] <= cXforBox3OnPlasticBelt_max AND (aBoxY[2] - aBoxY[3]) <= (cBoxWidth + 1))
						AND NOT (aBoxX[4] > (cXforBox4OnPlasticBelt_min + 20) AND aBoxX[4] <= cXforBox4OnPlasticBelt_max AND (aBoxY[2] - aBoxY[4]) <= (cBoxWidth + 1));
						
	aBoxPlasticFree[3] := 	NOT (aBoxX[1] > (cXforBox1OnPlasticBelt_min + 20) AND aBoxX[1] <= cXforBox1OnPlasticBelt_max AND (aBoxY[3] - aBoxY[1]) <= (cBoxWidth + 1))
						AND NOT (aBoxX[2] > (cXforBox2OnPlasticBelt_min + 20) AND aBoxX[2] <= cXforBox2OnPlasticBelt_max AND (aBoxY[3] - aBoxY[2]) <= (cBoxWidth + 1))
						AND NOT (aBoxX[4] > (cXforBox4OnPlasticBelt_min + 20) AND aBoxX[4] <= cXforBox4OnPlasticBelt_max AND (aBoxY[3] - aBoxY[4]) <= (cBoxWidth + 1));
						
	aBoxPlasticFree[4] := 	NOT (aBoxX[1] > (cXforBox1OnPlasticBelt_min + 20) AND aBoxX[1] <= cXforBox1OnPlasticBelt_max AND (aBoxY[4] - aBoxY[1]) <= (cBoxWidth + 1))
						AND NOT (aBoxX[2] > (cXforBox2OnPlasticBelt_min + 20) AND aBoxX[2] <= cXforBox2OnPlasticBelt_max AND (aBoxY[4] - aBoxY[2]) <= (cBoxWidth + 1))
						AND NOT (aBoxX[3] > (cXforBox3OnPlasticBelt_min + 20) AND aBoxX[3] <= cXforBox3OnPlasticBelt_max AND (aBoxY[4] - aBoxY[3]) <= (cBoxWidth + 1));
					
// =========================================================
// 塑料分拣气缸移动塑料物料

	FOR nState := 1 TO 4 BY 1 DO
		IF bPlasticToWork AND aBoxPlasticMove[nState] AND aBoxPlasticFree[nState] THEN
			IF (fYPlastic - cMetalPlasticCylMovement) >= (cYMetalPlasticCylEndPos + cMetalPlasticCylMovement) THEN
				fYPlastic := fYPlastic - cMetalPlasticCylMovement;
				
				IF (fYPlastic - aBoxY[nState]) <= cYMetalPlasticCylOnMainBelt THEN
					aBoxY[nState] := aBoxY[nState] - cMetalPlasticCylMovement;
				END_IF
				
			ELSIF fYPlastic = (cYMetalPlasticCylEndPos + cMetalPlasticCylMovement) AND (fYPlastic - aBoxY[nState]) <= cYMetalPlasticCylOnMainBelt THEN
				aBoxY[nState] := aBoxY[nState] - 2*cMetalPlasticCylMovement;
				
			ELSE
				aBoxPlasticMove[nState] := FALSE;
			END_IF
		END_IF	
	END_FOR

// =========================================================
END_METHOD

METHOD PRIVATE ErrorMessages
VAR_INPUT
END_VAR
// =========================== 错误信息 ==============================

	// 正位气缸错误条数以及信息
	IF bClampError THEN
		nMessages 			:= nMessages + 1;
		sMessageClamp 		:= CONCAT('Error of clamp cylinder: ', sClampErrMsg);	
	ELSE
		sMessageClamp 		:= '';
	END_IF
	
	// 金属分拣气缸错误条数以及信息
	IF bMetalCylError THEN
		nMessages 			:= nMessages + 1;
		sMessageMetalCyl 	:= CONCAT('Error of metal cylinder: ', sMetalErrMsg);
	ELSE
		sMessageMetalCyl 	:= '';
	END_IF
	
	// 塑料分拣气缸错误条数以及信息
	IF bPlasticCylError THEN
		nMessages 			:= nMessages + 1;
		sMessagePlasticCyl 	:= CONCAT('Error of plastic cylinder: ', sPlasticErrMsg);
	ELSE
		sMessagePlasticCyl 	:= '';
	END_IF
	
// =========================================================
END_METHOD

METHOD PRIVATE LastBox
VAR_INPUT
END_VAR
// =========================================================
// 检查输送皮带当中第几号物料在运输当中
	
	IF 		(aBoxX[1] >= (cXforAllBoxesStartPosMainBelt + 1*cBoxWidth - 0.05))
	AND		(aBoxX[1] < (cXforAllBoxesStartPosMainBelt + 2*cBoxWidth - 1.5)) AND (aBoxY[1] = 0) THEN
		nLastBox := 1;
		
	ELSIF 	(aBoxX[2] >= (cXforAllBoxesStartPosMainBelt + 2*cBoxWidth - 0.05))
	AND 	(aBoxX[2] < (cXforAllBoxesStartPosMainBelt + 3*cBoxWidth - 1.5)) AND (aBoxY[2] = 0) THEN
		nLastBox := 2;	
		
	ELSIF 	(aBoxX[3] >= (cXforAllBoxesStartPosMainBelt + 3*cBoxWidth - 0.05))
	AND 	(aBoxX[3] < (cXforAllBoxesStartPosMainBelt + 4*cBoxWidth - 1.5)) AND (aBoxY[3] = 0) THEN
		nLastBox := 3;	
		
	ELSIF 	(aBoxX[4] >= cXforAllBoxesStartPosMainBelt + 4*cBoxWidth - 0.05)
	AND 	(aBoxX[4] < (cXforAllBoxesStartPosMainBelt + 5*cBoxWidth - 1.5)) AND (aBoxY[4] = 0) THEN
		nLastBox := 4;	
		
	ELSE
		nLastBox := 0;
	END_IF		

// =========================================================
END_METHOD

METHOD PRIVATE Metal_Plastic_Cyl
VAR_INPUT
END_VAR
// =========================================================
// 移动金属分拣气缸
	
	IF bMetalToWork THEN
		IF NOT (aBoxMetalMove[1] OR aBoxMetalMove[2] OR aBoxMetalMove[3] OR aBoxMetalMove[4]) THEN
			IF ((fYMetal - cMetalPlasticCylMovement) >= cYMetalPlasticCylEndPos) THEN
				fYMetal := fYMetal - cMetalPlasticCylMovement;
			END_IF
			
		ELSE
			FOR nState := 1 TO 4 BY 1 DO
				IF aBoxMetalMove[nState] THEN
					IF ((fYMetal - cMetalPlasticCylMovement) >= (aBoxY[nState] - cYMetalPlasticCylOnMainBelt - 0.1))
					AND ((fYMetal - cMetalPlasticCylMovement) >= cYMetalPlasticCylEndPos) THEN
						fYMetal := fYMetal - cMetalPlasticCylMovement;
					END_IF
				END_IF
			END_FOR
		END_IF
		
	ELSE
		IF ((fYMetal + cMetalPlasticCylMovement) < cYMetalPlasticCylStartPos) THEN
			fYMetal := fYMetal + cMetalPlasticCylMovement;
		ELSE
			fYMetal := cYMetalPlasticCylStartPos;
		END_IF
	END_IF

// =========================================================
// 检测物料与金属分拣气缸的位置，判断物料是否正在被金属分拣气缸分拣，是否撞机
	
	IF (fYMetal < (cYMetalPlasticCylOnMainBelt + 0.1)) AND (fYMetal > (cYMetalPlasticCylOnMainBelt - 0.1)) AND bMetalToWork THEN
		FOR nState := 1 TO 4 BY 1 DO
			IF (aBoxY[nState] >= cYforAllBoxesOnMainBelt) THEN

				IF (aBoxX[nState] > (cXforAllBoxesCorrectPushMetalCyl_min + cBoxWidth*nState))
				AND (aBoxX[nState] <= (cXforAllBoxesCorrectPushMetalCyl_max + cBoxWidth*nState)) THEN
					aBoxMetalMove[nState] := TRUE;
				END_IF
				
				IF ((aBoxX[nState] > (cXforAllBoxesIncorrectPushMetalCyl_min + cBoxWidth*nState)
						AND aBoxX[nState] <= (cXforAllBoxesCorrectPushMetalCyl_min + cBoxWidth*nState))
					OR (aBoxX[nState] > (cXforAllBoxesCorrectPushMetalCyl_max + cBoxWidth*nState)
						AND aBoxX[nState] < (cXforAllBoxesIncorrectPushMetalCyl_max + cBoxWidth*nState)))
				AND NOT bStopped THEN
					bAccident := TRUE;
				END_IF
				
			END_IF
		END_FOR
	END_IF

// =========================================================
// =========================================================
// 移动塑料分拣气缸
	
	IF bPlasticToWork THEN
		IF NOT (aBoxPlasticMove[1] OR aBoxPlasticMove[2] OR aBoxPlasticMove[3] OR aBoxPlasticMove[4]) THEN
			IF ((fYPlastic - cMetalPlasticCylMovement) >= cYMetalPlasticCylEndPos) THEN
				fYPlastic := fYPlastic - cMetalPlasticCylMovement;
			END_IF
			
		ELSE
			FOR nState := 1 TO 4 BY 1 DO
				IF aBoxPlasticMove[nState] THEN
					IF ((fYPlastic - cMetalPlasticCylMovement) >= (aBoxY[nState] - cYMetalPlasticCylOnMainBelt - 0.1))
					AND ((fYPlastic - cMetalPlasticCylMovement) >= cYMetalPlasticCylEndPos) THEN
						fYPlastic := fYPlastic - cMetalPlasticCylMovement;
					END_IF
				END_IF
			END_FOR
		END_IF
		
	ELSE
		IF ((fYPlastic + cMetalPlasticCylMovement) < cYMetalPlasticCylStartPos) THEN
			fYPlastic := fYPlastic + cMetalPlasticCylMovement;
		ELSE
			fYPlastic := cYMetalPlasticCylStartPos;
		END_IF
	END_IF

// =========================================================
// 检测物料与塑料分拣气缸的位置，判断物料是否正在被塑料分拣气缸分拣，是否撞机
		
	IF ((aBoxX[1] > (cXforAllBoxesLastPossiblePosMainBelt + 1*cBoxWidth))
		OR (aBoxX[2] > (cXforAllBoxesLastPossiblePosMainBelt + 2*cBoxWidth))
		OR (aBoxX[3] > (cXforAllBoxesLastPossiblePosMainBelt + 3*cBoxWidth))
		OR (aBoxX[4] > (cXforAllBoxesLastPossiblePosMainBelt + 4*cBoxWidth)))
	AND NOT bStopped THEN
		bAccident := TRUE;
	END_IF
		
	IF (fYPlastic < (cYMetalPlasticCylOnMainBelt + 0.1)) AND (fYPlastic > (cYMetalPlasticCylOnMainBelt - 0.1)) AND bPlasticToWork THEN
		FOR nState := 1 TO 4 BY 1 DO
			IF aBoxY[nState] >= cYforAllBoxesOnMainBelt THEN
				
				IF (aBoxX[nState] > (cXforAllBoxesCorrectPushPlasticCyl_min + cBoxWidth*nState))
				AND (aBoxX[nState] <= (cXforAllBoxesCorrectPushPlasticCyl_max + cBoxWidth*nState)) THEN
					aBoxPlasticMove[nState] := TRUE;
				END_IF
				
				IF (aBoxX[nState] > (cXforAllBoxesIncorrectPushPlasticCyl_min + cBoxWidth*nState))
				AND (aBoxX[nState] <= (cXforAllBoxesCorrectPushPlasticCyl_min + cBoxWidth*nState))
				AND NOT bStopped THEN
					bAccident := TRUE;
				END_IF	
				
			END_IF
		END_FOR
	END_IF

// =========================================================
END_METHOD

PROPERTY P_ArrChangeColor : ARRAY [1..4] OF BOOL
GET
P_ArrChangeColor	:= ArrChangeColor;
END_GET
END_PROPERTY

PROPERTY P_ArrfBoxX : ARRAY [1..4] OF LREAL
GET
P_ArrfBoxX	:= ABoxX;
END_GET
END_PROPERTY

PROPERTY P_ArrfBoxY : ARRAY [1..4] OF LREAL
GET
P_ArrfBoxY	:= ABoxY;
END_GET
END_PROPERTY

PROPERTY P_fYBarrier : LREAL
GET
P_fYBarrier	:= fYBarrier;
END_GET
END_PROPERTY

PROPERTY P_fYClamp : LREAL
GET
P_fYClamp	:= fYClamp;
END_GET
END_PROPERTY

PROPERTY P_fYMetal : LREAL
GET
P_fYMetal	:= fYMetal;
END_GET
END_PROPERTY

PROPERTY P_fYPlastic : LREAL
GET
P_fYPlastic	:= fYPlastic;
END_GET
END_PROPERTY

METHOD PRIVATE RandomColor
VAR_INPUT
END_VAR
// =========================================================

// 随机数（0..1）生成器
RandomGenerator(Seed:= 1 , Num=> RandomNumber);

// 随机BOOL变量生成器
IF RandomNumber >0.5 THEN
	bRandomChangeColor	:= TRUE;
ELSE
	bRandomChangeColor	:= FALSE;
END_IF

// =========================================================
END_METHOD

METHOD PRIVATE Reset
VAR_INPUT
END_VAR
// ========================== 复位Visu相关变量 ===============================
	
	// 气缸按钮
	bButtonClampToWorkOut 		:= FALSE;
	bButtonBarrierToWorkOut 	:= FALSE;
	bButtonMetalToWorkOut 		:= FALSE;
	bButtonPlasticToWorkOut 	:= FALSE;
	
	// 轴控按钮
	bButtonMainBwOut 			:= FALSE;
	bButtonMainFwOut 			:= FALSE;
	bButtonMetalBwOut 			:= FALSE;
	bButtonMetalFwOut 			:= FALSE;
	bButtonPlasticBwOut			:= FALSE;
	bButtonPlasticFwOut			:= FALSE;
	
	// 模式以及状态按钮
	bButtonStartOut 			:= FALSE;
	bButtonStopOut 				:= FALSE;
	bButtonResetOut 			:= FALSE;
	bButtonComprAirOut 			:= FALSE;
	bButtonManuOut 				:= FALSE;
	bButtonAutoOut 				:= FALSE;
	bButtonSemiOut 				:= FALSE;
	bButtonMaintenanceOut		:= FALSE;
	
	// 物料状态的相关变量
	FOR nState := 1 TO 4 BY 1 DO
		aBoxX[nState] 			:= 0;
		aBoxY[nState] 			:= 0;
		
		aBoxMetalMove[nState] 	:= FALSE;
		aBoxPlasticMove[nState]	:= FALSE;
		aBoxMainBelt[nState]	:= FALSE;
		aBoxMetalBelt[nState] 	:= FALSE;
		aBoxPlasticBelt[nState]	:= FALSE;
	END_FOR
	
	// 事故标志位
	bAccident := FALSE;

// =========================================================
END_METHOD

END_FUNCTION_BLOCK
